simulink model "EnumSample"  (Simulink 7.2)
settings: Solver=ode45  StartTime=0.0  StopTime=10.0  RelTol=1e-3
undefined symbols (not defined in the file or in its folder): ControlModeEnum, Enum, ErrorCodeEnum, FeedModeEnum

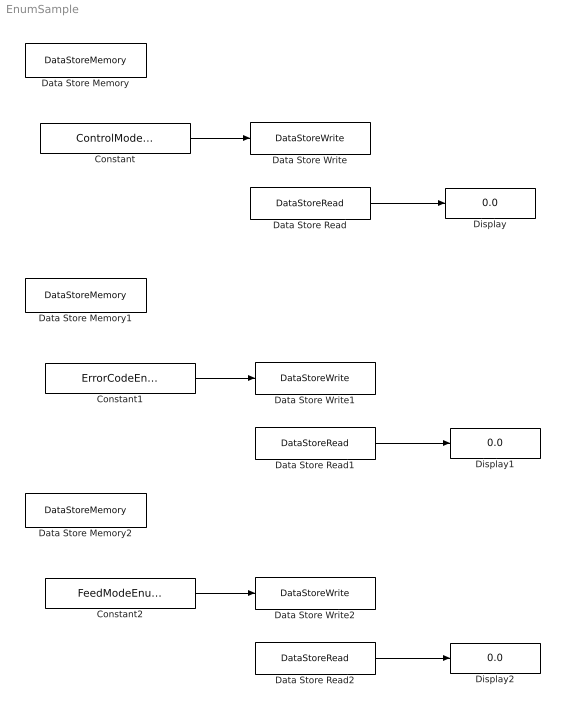
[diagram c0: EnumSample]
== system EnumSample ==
  Constant : Constant  Value=ControlModeEnum.IDLE  OutDataTypeMode=Specify via dialog  OutDataType=Enum: ControlModeEnum  ConRadixGroup=Best Precision: Vector-wise  OutDataTypeStr=Enum: ControlModeEnum
  Constant1 : Constant  Value=ErrorCodeEnum.ERROR_001  OutDataTypeMode=Specify via dialog  OutDataType=Enum:ErrorCodeEnum  ConRadixGroup=Best Precision: Vector-wise  OutDataTypeStr=Enum:ErrorCodeEnum
  Constant2 : Constant  Value=FeedModeEnum.PAPERFEED  OutDataTypeMode=Specify via dialog  OutDataType=Enum: FeedModeEnum  ConRadixGroup=Best Precision: Vector-wise  OutDataTypeStr=Enum: FeedModeEnum
  Data Store Memory : DataStoreMemory  DataStoreName=ControlMode  ReadBeforeWriteMsg=warning  WriteAfterWriteMsg=warning  WriteAfterReadMsg=warning  InitialValue=ControlModeEnum.IDLE  DataType=Specify via dialog  OutDataType=Enum: ControlModeEnum  OutDataTypeStr=Enum: ControlModeEnum
  Data Store Memory1 : DataStoreMemory  DataStoreName=ErrorCode  ReadBeforeWriteMsg=warning  WriteAfterWriteMsg=warning  WriteAfterReadMsg=warning  InitialValue=ErrorCodeEnum.NO_ERROR  DataType=Specify via dialog  OutDataType=Enum: ErrorCodeEnum  OutDataTypeStr=Enum: ErrorCodeEnum
  Data Store Memory2 : DataStoreMemory  DataStoreName=FeedMode  ReadBeforeWriteMsg=warning  WriteAfterWriteMsg=warning  WriteAfterReadMsg=warning  InitialValue=FeedModeEnum.IDLE  DataType=Specify via dialog  OutDataType=Enum: FeedModeEnum  OutDataTypeStr=Enum: FeedModeEnum
  Data Store Read : DataStoreRead  DataStoreName=ControlMode  SampleTime=-1
  Data Store Read1 : DataStoreRead  DataStoreName=ErrorCode  SampleTime=-1
  Data Store Read2 : DataStoreRead  DataStoreName=FeedMode  SampleTime=-1
  Data Store Write : DataStoreWrite  DataStoreName=ControlMode  SampleTime=-1
  Data Store Write1 : DataStoreWrite  DataStoreName=ErrorCode  SampleTime=-1
  Data Store Write2 : DataStoreWrite  DataStoreName=FeedMode  SampleTime=-1
  Display : Display
  Display1 : Display
  Display2 : Display
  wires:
  Constant/1 -> Data Store Write/1
  Data Store Read/1 -> Display/1
  Constant1/1 -> Data Store Write1/1
  Data Store Read1/1 -> Display1/1
  Constant2/1 -> Data Store Write2/1
  Data Store Read2/1 -> Display2/1
